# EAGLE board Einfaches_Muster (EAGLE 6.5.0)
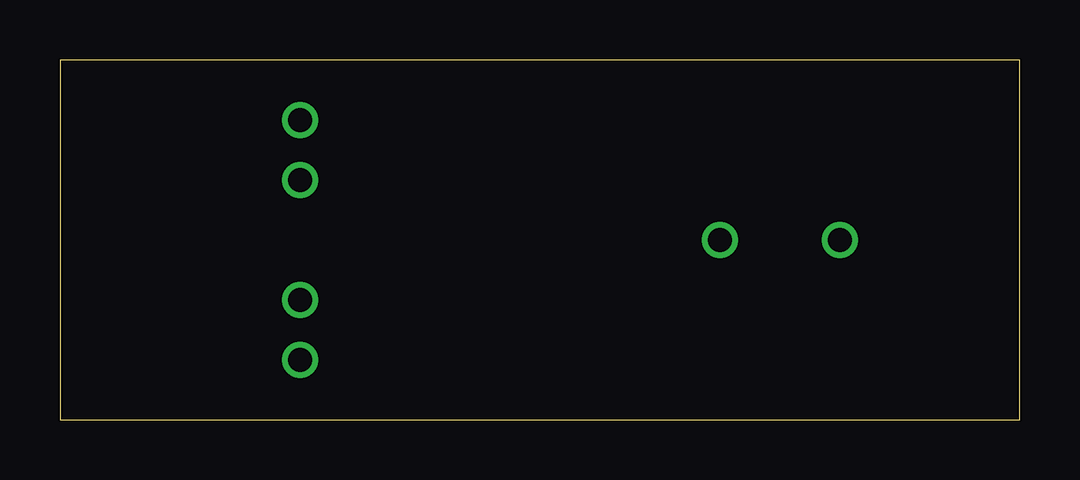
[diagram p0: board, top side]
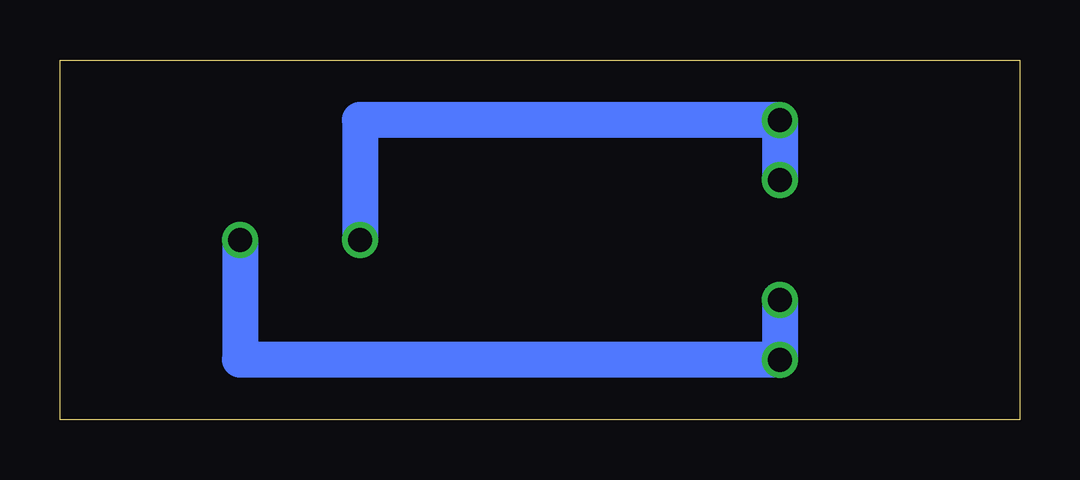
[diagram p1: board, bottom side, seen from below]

Size 40 x 15 mm. Coordinates in mm from the lower left corner, seen from the top.
Outline: 0,0 40,0 40,15 0,15 0,0
Copper layers (1*16): Top 0.035mm / dielectric 1.5mm / Bottom 0.035mm
Design rules "default": minimum track width 10mil, minimum drill 24mil, track to track 8mil, track to pad 8mil, pad to pad 8mil, via to via 8mil, smd to smd 8mil, copper to edge 40mil, drill to drill 8mil, minimum pad ring 10mil, minimum via ring 8mil, stop-mask expansion 4mil, vias tented up to drill 0mil, thermal gap 10mil

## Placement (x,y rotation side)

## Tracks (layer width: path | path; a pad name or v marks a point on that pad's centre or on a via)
S$1  (via drill 1)
  Bottom 1.5: v32.5,7.5 32.5,2.5 v10,2.5 v10,5
S$3  (via drill 1)
  Bottom 1.5: v10,10 v10,12.5 27.5,12.5 27.5,7.5
S$5  (via drill 1)
  other vias: 27.5,7.5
